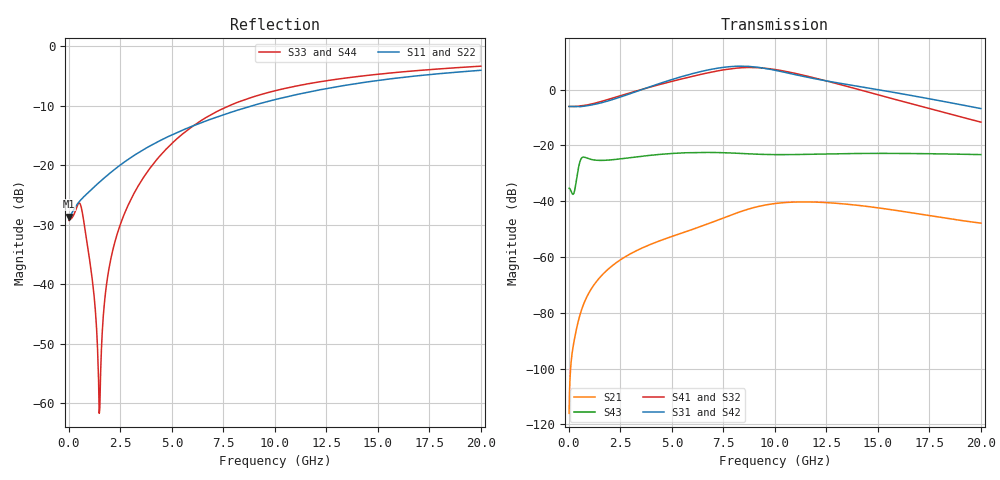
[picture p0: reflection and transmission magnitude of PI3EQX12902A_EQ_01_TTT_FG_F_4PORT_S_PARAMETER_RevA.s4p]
! NPort=4 DATA=2000 NOISE=0 GROUPDELAY=0 COMPLEX_DATAFORMAT=POLAR
! NumOfBlock=1 NumOfParam=0
! .MODEL Smodel S TSTONEFILE=PI3EQX12902A_EQ_01_TTT_FG_F_4PORT_S_PARAMETER_RevA.s4p TYPE=S
!  -- The above .MODEL line can be used for the S element in the netlist.
! The s parameter is extracted from the linear redriver, it is not bi-directional; only s(4,1)s(4,2) and s(3,1)s(3,2)
! should be the insertion loss
!Port definition:
!Port1 = input+
!Port2 = input-
!Port3 = output+
!Port4 = output-
# Hz S MA R  50
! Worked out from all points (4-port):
!   2000 points, 10 MHz to 20 GHz, reference 50 ohm
!   strongest paths, dB at 10 MHz, 5.01 GHz, 10.01 GHz, 15.01 GHz, 20 GHz:
!     S31: -6.0, 3.6, 6.9, 0.0, -6.8
!     S42: -6.0, 3.5, 6.8, -0.3, -7.0
!     S41: -6.0, 3.0, 7.2, -1.9, -11.7
!     S32: -6.0, 3.0, 7.2, -1.9, -11.8
!     S43: -35.3, -22.9, -23.3, -22.9, -23.3
!     S21: -116.0, -52.6, -40.8, -42.4, -47.9
!   lowest |S11| = -28.6 dB at 10 MHz (marker M1), VSWR 1.08, Z = 46.4 - j0.0607 ohm
!   |S11| at or under -10 dB: start of sweep to 8.91 GHz
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1e7  0.03704 -179.0  1.583e-06 51.7  0 0.0  0 0.0
     1.583e-06 51.7  0.03704 -179.0  0 0.0  0 0.0
     0.4985 -0.0  0.4985 180.0  0.03429 6.0  0.01709 -177.1
     0.4985 180.0  0.4985 -0.0  0.01709 -177.1  0.03429 6.0
1.49e9  0.07219 -133.4  0.0004252 115.8  3.742e-09 177.1  5.624e-09 -173.9
        0.0004252 115.8  0.07219 -133.4  5.626e-09 -173.8  3.743e-09 177.2
        0.57 8.7  0.6034 -177.6  0.0008858 -60.3  0.05389 -174.9
        0.6016 -177.7  0.5699 8.4  0.05389 -174.8  0.0009453 -62.8
6.08e9  0.2159 -112.2  0.003199 84.8  1.763e-06 -26.2  1.114e-06 84.5
        0.003202 84.8  0.2159 -112.2  1.121e-06 84.7  1.758e-06 -26.1
        1.967 -43.7  1.759 108.4  0.2166 -47.3  0.07412 143.8
        1.757 108.5  1.936 -44.3  0.07451 143.9  0.216 -47.3
7.78e9  0.275 -112.0  0.005476 71.3  5.788e-06 -76.4  3.74e-06 41.1
        0.005494 71.3  0.275 -112.0  3.778e-06 41.1  5.778e-06 -76.3
        2.57 -89.7  2.342 60.3  0.3157 -64.0  0.07286 126.1
        2.339 60.3  2.527 -90.2  0.07333 126.0  0.315 -63.9
9.34e9  0.3323 -113.3  0.008229 45.4  1.136e-05 -123.0  8.383e-06 -10.8
        0.008268 45.2  0.3323 -113.3  8.476e-06 -11.0  1.135e-05 -122.8
        2.462 -137.2  2.449 6.9  0.3931 -76.7  0.06879 114.3
        2.447 7.0  2.417 -137.7  0.06917 114.1  0.3927 -76.6
1.17e10  0.4143 -116.8  0.009646 1.5  2.009e-05 -176.6  1.491e-05 -86.4
         0.009687 1.1  0.4143 -116.8  1.506e-05 -86.8  2.006e-05 -176.5
         1.629 169.8  1.69 -65.3  0.4863 -91.3  0.06923 100.9
         1.695 -65.1  1.59 169.4  0.06936 100.7  0.4865 -91.2
2e10  0.6274 -131.5  0.004152 -68.8  4.492e-05 49.7  1.718e-05 108.0
      0.004047 -69.3  0.6274 -131.5  1.733e-05 107.1  4.476e-05 50.0
      0.4572 46.1  0.2574 138.6  0.6794 -119.6  0.06846 46.2
      0.2613 138.3  0.4465 46.6  0.06841 46.2  0.6798 -119.6
